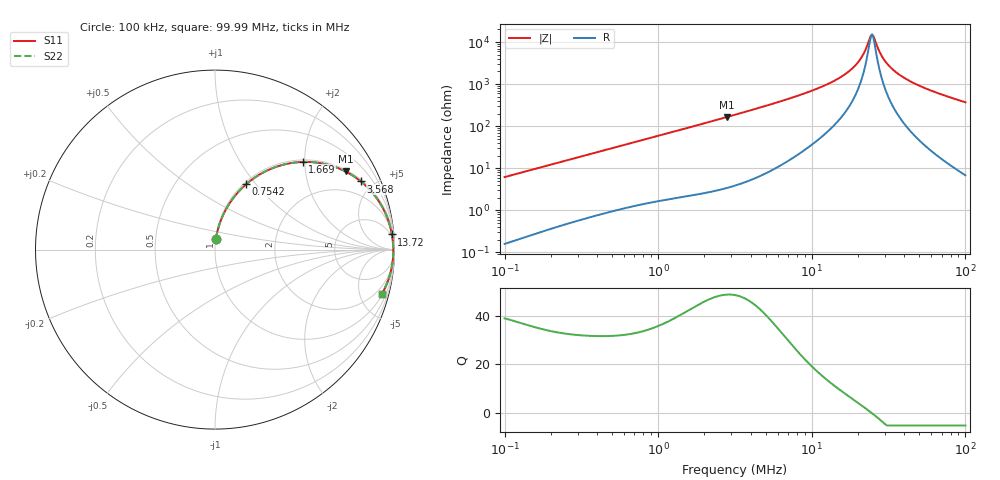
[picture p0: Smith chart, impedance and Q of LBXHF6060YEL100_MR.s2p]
! LBXHF6060YEL100_MR  S-PARAMETER MODEL  ( General Type )
! Model Generated by TAIYO YUDEN Corporation (http://www.ty-top.com)
! Version 1.0
! TAIYO YUDEN Control No. 200120NI43SB-FBB
! Copyright(c) 2020 TAIYO YUDEN CO.,LTD. All Rights Reserved.
! Product Description (link to TY-COMPAS)
! https://ds.yuden.co.jp/TYCOMPAS/or/detail?pn=LBXHF6060YEL100MMR&u=M
! Products Name : Inductors
! Characteristics :
!  Inductance : 10 uH , SRF(min) : 16 MHz , DC Resistance(max) : 0.06 Ohm
!  Rated Current : Saturation :4000 mA , Temp Rise : 1800 mA
!  Case Size : 6.0 x 6.0 / 0.236 x 0.236 [mm/inch] , Thickness : 4.5 / 0.177 [mm/inch]
!  (Conditions: Temperature = 25 degC , DC Bias Current/Voltage = 0A / 0V)
! External Node Assignments :
!  1  o---GGG---o  2
! GND o---------o GND
! Frequency Range : 0.1MHz  -  99.992428MHz  [ 402 STEP ]
# MHz S RI R 50
! Freq[MHz].  S11 Real  S11 Imag  S21 Real  S21 Imag  S12 Real  S12 Imag  S22 Real  S22 Imag
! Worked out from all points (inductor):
!   401 points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, 100 kHz to 99.99 MHz, reference 50 ohm
!   read as one part in series: L = 9.77 uH near 103.5 kHz
!   highest Q = 48.6 at 2.802 MHz (marker M1), where L = 9.37 uH
!   self-resonance near 24.26 MHz
!   S11 on the Smith chart (normalised r, x): 100 kHz: 1.00, +0.12; 754.2 kHz: 1.03, +0.89; 1.669 MHz: 1.05, +1.95; 3.568 MHz: 1.09, +4.23; 13.72 MHz: 3, +23; 99.99 MHz: 1.14, -7.40
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0.1  0.00534 0.0611  0.9947 -0.0611  0.9947 -0.0611  0.00534 0.0611
0.318049  0.0408 0.1828  0.9592 -0.1828  0.9592 -0.1828  0.0408 0.1828
0.754207  0.1733 0.3637  0.8267 -0.3637  0.8267 -0.3637  0.1733 0.3637
1.011554  0.2672 0.4288  0.7328 -0.4288  0.7328 -0.4288  0.2672 0.4288
1.669116  0.4888 0.4884  0.5112 -0.4884  0.5112 -0.4884  0.4888 0.4884
2.802103  0.7271 0.4353  0.2729 -0.4353  0.2729 -0.4353  0.7271 0.4353
3.162158  0.7725 0.409  0.2275 -0.409  0.2275 -0.409  0.7725 0.409
3.568478  0.8125 0.3799  0.1875 -0.3799  0.1875 -0.3799  0.8125 0.3799
5.688277  0.9183 0.2606  0.0817 -0.2606  0.0817 -0.2606  0.9183 0.2606
10.05722  0.9732 0.1374  0.0268 -0.1374  0.0268 -0.1374  0.9732 0.1374
13.72387  0.9854 0.0845  0.0146 -0.0845  0.0146 -0.0845  0.9854 0.0845
16.59494  0.9897 0.0557  0.0103 -0.0557  0.0103 -0.0557  0.9897 0.0557
19.38541  0.9919 0.0334  0.00808 -0.0334  0.00808 -0.0334  0.9919 0.0334
21.50178  0.9928 0.019  0.00715 -0.019  0.00715 -0.019  0.9928 0.019
23.84921  0.9934 0.00462  0.00663 -0.00462  0.00663 -0.00462  0.9934 0.00462
24.68731  0.9934 -0.000152  0.00655 0.000152  0.00655 0.000152  0.9934 -0.000152
25.55487  0.9935 -0.00493  0.00651 0.00493  0.00651 0.00493  0.9935 -0.00493
28.83852  0.9933 -0.0218  0.00675 0.0218  0.00675 0.0218  0.9933 -0.0218
31.98693  0.9926 -0.0365  0.00743 0.0365  0.00743 0.0365  0.9926 -0.0365
38.01646  0.9903 -0.062  0.00968 0.062  0.00968 0.062  0.9903 -0.062
48.41396  0.9843 -0.1006  0.0157 0.1006  0.0157 0.1006  0.9843 -0.1006
99.99243  0.928 -0.2495  0.072 0.2495  0.072 0.2495  0.928 -0.2495
